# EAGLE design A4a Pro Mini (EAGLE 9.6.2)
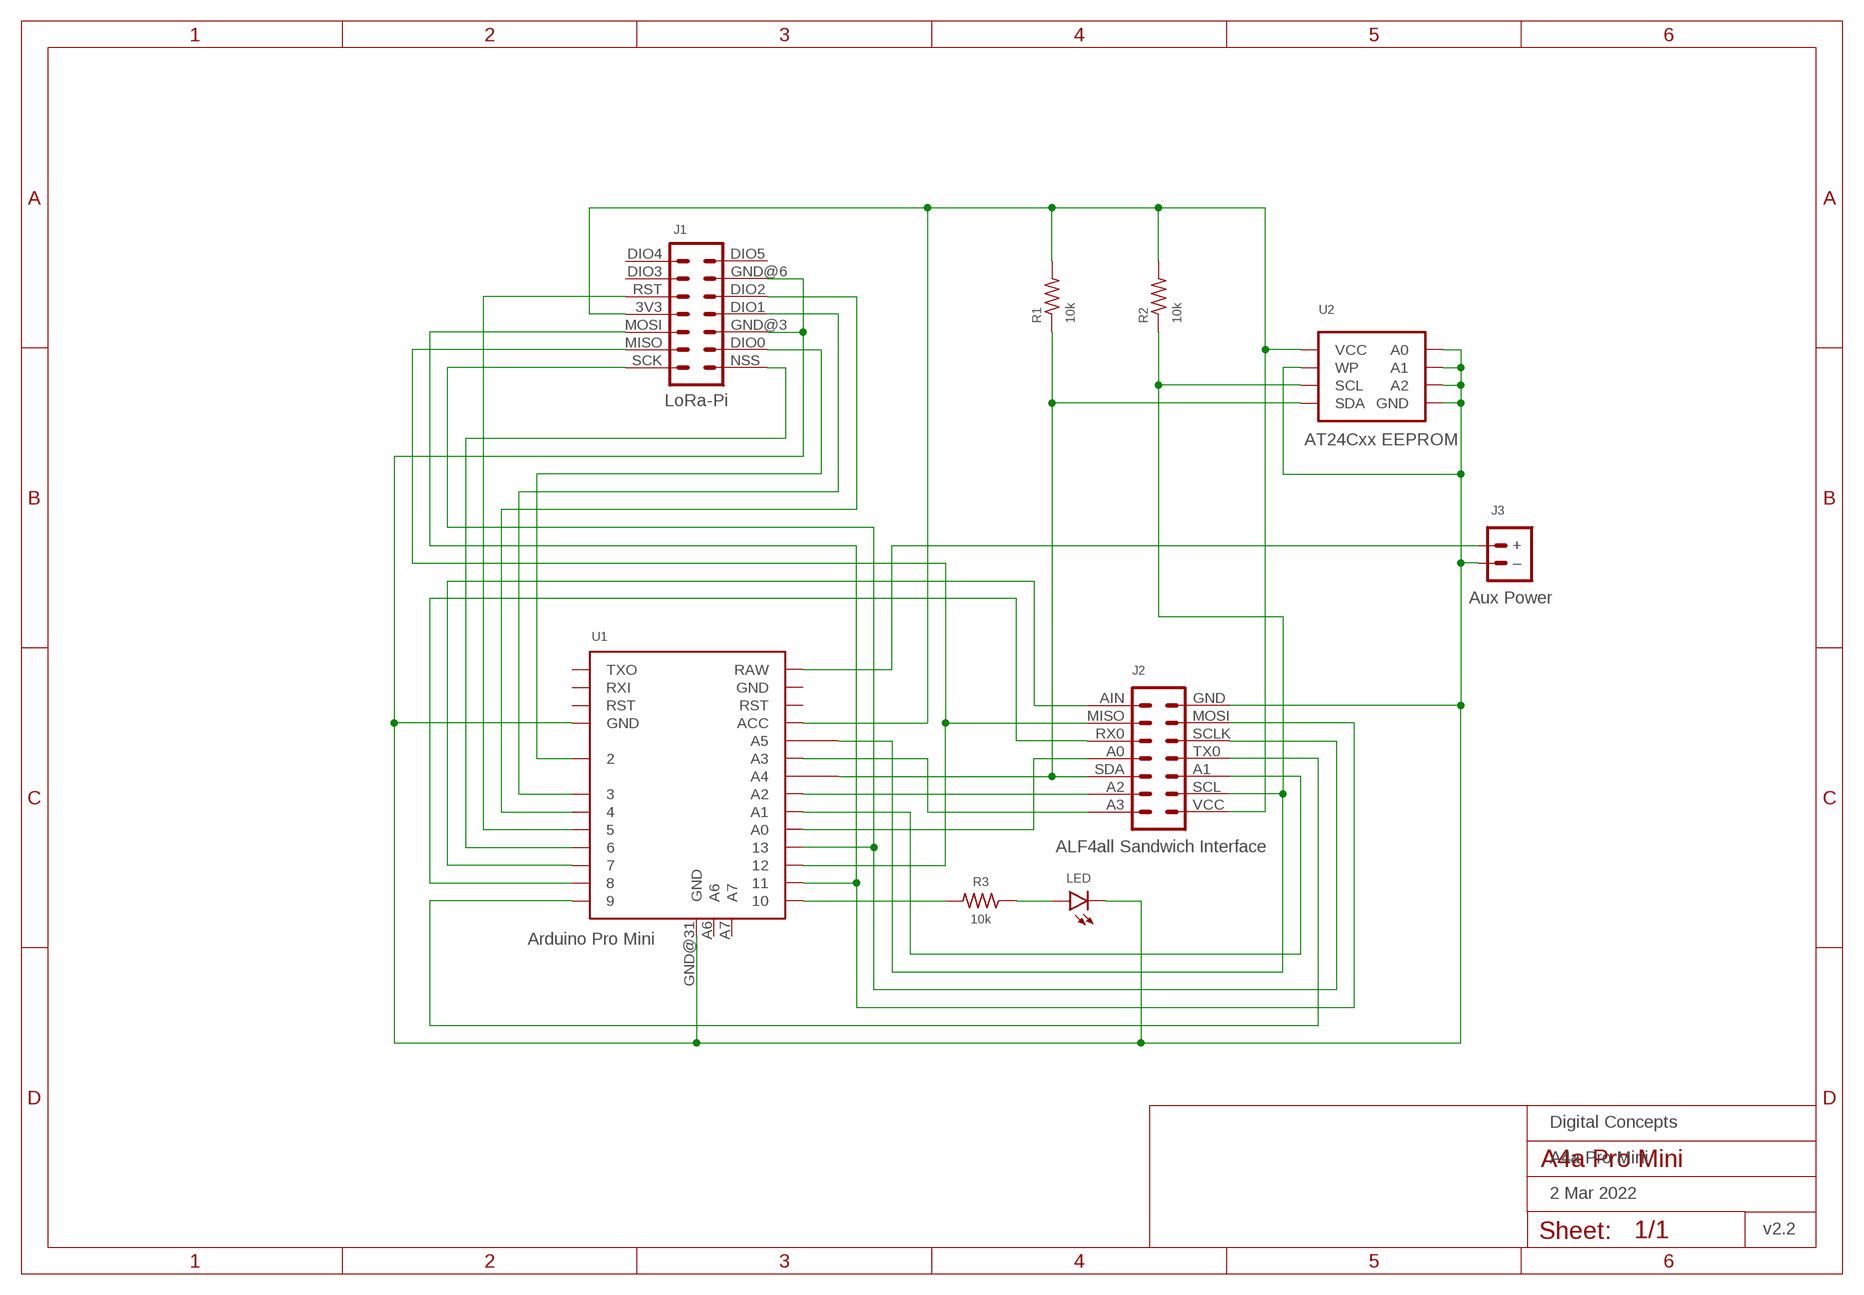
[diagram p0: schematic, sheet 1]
FRAME1 (A4L-LOC): DATE: 2 Mar 2022; OWNER: Digital Concepts; TITLE: A4a Pro Mini; VERSION: v2.2

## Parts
J1  LoRa-Pi  RFM95W-PI-HEADER  [RFM95W-PI]
J2  ALF4all Sandwich Interface  HEADER-2X7-ALF4ALL-PROCESSOR-B  [CONN_2X7-ALF4ALL-PROCESSOR-B]
J3  Aux Power  JST-PH2.0-2-MALE-HORIZONTALJST-PTH-2  [JST-PH2.0-2-HORIZONTAL]
LED  LEDCHIP-LED0805  [CHIP-LED0805]
R1  10k  RESISTORR0805  [R0805]
R2  10k  RESISTORR0805  [R0805]
R3  10k  RESISTORR0805  [R0805]
U1  Arduino Pro Mini  ARDUINO-PRO-MINI-35  [ARDUINO-PRO-MINI-35]
U2  AT24Cxx EEPROM  AT24CXX-EEPROM  [SOP-8]

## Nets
GND: J1.GND@3 J1.GND@6 J2.GND J3.-(–) LED.C U1.GND@22(GND) U1.GND@31(GND) U2.P$1(A0) U2.P$2(A1) U2.P$3(A2) U2.P$4(GND) U2.P$7(WP)
N$1: J2.A0 U1.A0
N$2: J2.A1 U1.A1
N$3: J2.A2 U1.A2
N$4: J2.A3 U1.A3
N$5: J3.+ U1.RAW
N$6: J1.SCK J2.SCLK U1.13
N$7: J2.RX0 U1.8
N$9: J2.AIN U1.7
N$10: J2.SDA R1.1 U1.A4 U2.P$5(SDA)
N$11: J2.SCL R2.1 U1.A5 U2.P$6(SCL)
N$12: J1.MISO J2.MISO U1.12
N$13: J1.MOSI J2.MOSI U1.11
N$14: J2.TX0 U1.9
N$15: J1.NSS U1.6
N$16: J1.RST U1.5
N$17: J1.DIO2 U1.4
N$18: J1.DIO1 U1.3
N$19: J1.DIO0 U1.2
N$20: R3.2 U1.10
N$21: LED.A R3.1
VCC: J1.3V3 J2.VCC R1.2 R2.2 U1.ACC U2.P$8(VCC)
Unconnected: J1.DIO3 J1.DIO4 J1.DIO5 U1.A6 U1.A7 U1.GND@11(GND) U1.RST@10(RST) U1.RST@21(RST) U1.RXI@20(RXI) U1.TXO@19(TXO)

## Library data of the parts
J1 = digitalconcepts:RFM95W-PI-HEADER: RFM95W LoRa Wireless Transceiver Raspberry Pi Daughter Board
J2 = digitalconcepts:HEADER-2X7-ALF4ALL-PROCESSOR-B: ALF4all 'Sandwich' Processor (Bottom) 2x7 Pin Header Header soldered to underside of PCB
J3 = digitalconcepts:JST-PH2.0-2-MALE-HORIZONTAL: Multi connection point. Often used as Generic Header-pin footprint for 0.1 inch spaced/style header connections; PROD_ID: CONN-09863; SKU: PRT-09914
LED = digitalconcepts:LED: LED
R1-R3 = digitalconcepts:RESISTOR: Resistor; SPICEPREFIX: R
U1 = digitalconcepts:ARDUINO-PRO-MINI-35: Arduino Pro Mini 35-pin Clone
U2 = digitalconcepts:AT24CXX-EEPROM: AT24Cxx EEPROM SOP-8

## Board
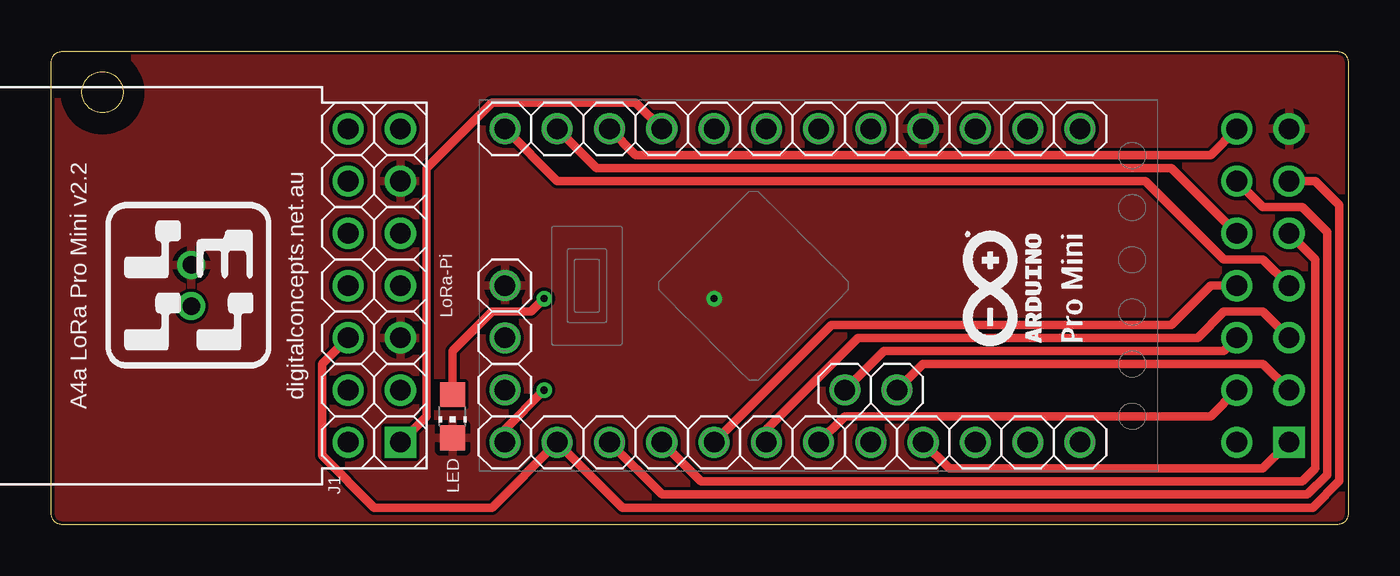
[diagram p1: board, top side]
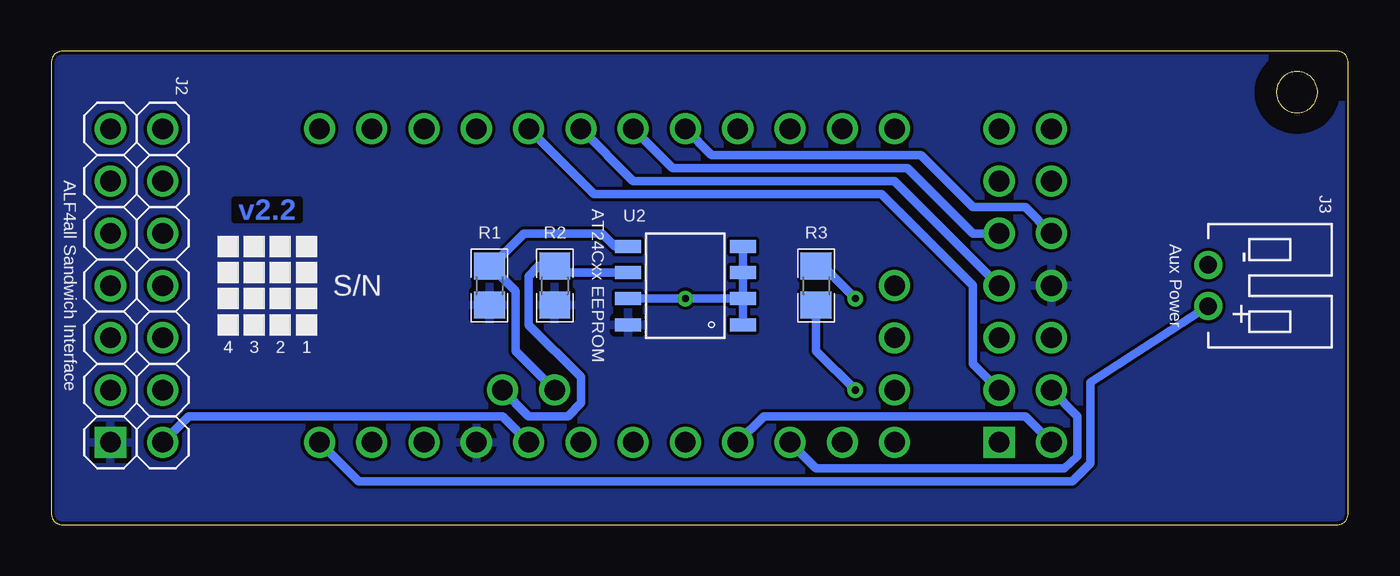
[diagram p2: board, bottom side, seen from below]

Size 63 x 23 mm. Coordinates in mm from the lower left corner, seen from the top.
Outline: 179 segments
Copper layers (1*16): Top 0.035mm / dielectric 1.5mm / Bottom 0.035mm
Design rules "default *": minimum track width 6mil, minimum drill 0.35mm, track to track 6mil, track to pad 6mil, pad to pad 6mil, via to via 6mil, smd to smd 6mil, copper to edge 6mil, drill to drill 6mil, minimum pad ring 10mil, minimum via ring 8mil, stop-mask expansion 4mil, vias tented up to drill 0mil, thermal gap 10mil

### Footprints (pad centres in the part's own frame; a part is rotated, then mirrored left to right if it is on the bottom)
RFM95W-PI = drill 1 pad 1.524: 3V3 7.62,2.54; DIO0 2.54,0; DIO1 7.62,0; DIO2 10.16,0; DIO3 12.7,2.54; DIO4 15.24,2.54; DIO5 15.24,0; GND@3 5.08,0; GND@6 12.7,0; MISO 2.54,2.54; MOSI 5.08,2.54; RST 10.16,2.54; SCK 0,2.54 | drill 1 pad 1.524 square: NSS 0,0
CONN_2X7-ALF4ALL-PROCESSOR-B = drill 1 pad 1.524: A0 7.62,2.54; A1 5.08,0; A2 2.54,2.54; A3 0,2.54; AIN 15.24,2.54; GND 15.24,0; MISO 12.7,2.54; MOSI 12.7,0; RX0 10.16,2.54; SCL 2.54,0; SCLK 10.16,0; SDA 5.08,2.54; TX0 7.62,0 | drill 1 pad 1.524 square: VCC 0,0
JST-PH2.0-2-HORIZONTAL = drill 0.85: + 1,0; - -1,0
CHIP-LED0805 = smd 1.2 x 1.2: A 0,-1.05; C 0,1.05
R0805 = smd 1.3 x 1.5: 1 -0.95,0; 2 0.95,0
ARDUINO-PRO-MINI-35 = drill 1: 2 -15.24,17.78; 3 -15.24,15.24; 4 -15.24,12.7; 5 -15.24,10.16; 6 -15.24,7.62; 7 -15.24,5.08; 8 -15.24,2.54; 9 -15.24,0; 10 0,0; 11 0,2.54; 12 0,5.08; 13 0,7.62; A0 0,10.16; A1 0,12.7; A2 0,15.24; A3 0,17.78; A4 -2.54,16.51; A5 -2.54,19.05; A6 -5.08,0; A7 -2.54,0; ACC 0,20.32; GND@11 0,25.4; GND@22 -15.24,20.32; GND@31 -7.62,0; RAW 0,27.94; RST@10 0,22.86; RST@21 -15.24,22.86; RXI@20 -15.24,25.4; TXO@19 -15.24,27.94
SOP-8 = smd 0.635 x 1.27: P$1 -1.905,-2.794; P$2 -0.635,-2.794; P$3 0.635,-2.794; P$4 1.905,-2.794; P$5 1.905,2.794; P$6 0.635,2.794; P$7 -0.635,2.794; P$8 -1.905,2.794

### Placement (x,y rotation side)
J1  16.96,4 90 top
J2  60.14,4 90 top
J3  6.8,11.62 270 bottom
LED  19.5,5.27 180 top
R1  41.72,11.62 270 bottom
R2  38.55,11.62 270 bottom
R3  25.85,11.62 270 bottom
U1  22.04,4 270 top
U2  32.2,11.62 90 bottom

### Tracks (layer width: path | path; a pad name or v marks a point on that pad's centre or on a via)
$X1
  cutout Top: 2.48,23.05 arc180 2.48,18.98 arc180
$X10
  cutout Bottom: 2.48,23.05 arc180 2.48,18.98 arc180
GND  (via drill 0.35)
  Bottom 0.406: U2.P$2 U2.P$3 U2.P$4 | U2.P$2 U2.P$1 | U2.P$2 v32.2,10.98 U2.P$7
  pour Top: -2.09,25.59 65.22,25.59 65.22,-2.35 -2.09,-2.35
N$1
  Top 0.406: J2.A0 56.33,11.62 54.42,9.71 37.91,9.71 U1.A0
N$2
  Top 0.406: J2.A1 58.87,10.35 56.96,10.35 55.69,9.08 39.18,9.08 34.74,4.63 U1.A1
N$3
  Top 0.406: J2.A2 56.33,5.27 38.55,5.27 U1.A2
N$4
  Bottom 0.406: J2.A3 56.33,5.27 41.09,5.27 U1.A3
N$5
  Bottom 0.406: J3.+ 12.51,6.9 12.51,2.98 13.4,2.09 48.07,2.09 U1.RAW
N$6
  Top 0.406: J2.SCLK 61.41,12.89 61.41,2.73 60.77,2.09 31.56,2.09 U1.13
  Bottom 0.406: J1.SCK 15.69,5.27 28.39,5.27 U1.13
N$7
  Top 0.406: J2.RX0 54.42,17.33 26.48,17.33 U1.8
N$9
  Top 0.406: J2.AIN 56.33,17.97 28.39,17.97 U1.7
N$10
  Top 0.406: J2.SDA 56.96,8.44 40.45,8.44 U1.A4
  Bottom 0.406: U2.P$5 35.62,13.52 36.26,14.16 40.03,14.16 41.62,12.57 R1.1 41.67,12.57 40.45,11.35 40.45,8.44 U1.A4
N$11
  Top 0.406: J2.SCL 58.87,7.81 42.36,7.81 U1.A5
  Bottom 0.406: U1.A5 39.82,5.27 37.91,5.27 37.28,5.9 37.28,7.17 39.82,9.71 39.82,12.07 39.33,12.57 R2.1 38.23,12.25 U2.P$6
N$12
  Top 0.406: J2.MISO 58.87,15.43 60.77,15.43 61.99,14.21 61.99,2.42 61.02,1.46 29.66,1.46 U1.12
  Bottom 0.406: J1.MISO 13.15,5.27 13.15,3.31 13.78,2.73 25.85,2.73 U1.12
N$13
  Top 0.406: J2.MOSI 61.41,16.7 62.57,15.53 62.57,2.12 61.28,0.82 27.75,0.82 U1.11 21.4,0.82 15.69,0.82 13.15,3.36 13.15,7.81 J1.MOSI
N$14
  Top 0.406: J2.TX0 58.87,12.89 56.96,12.89 53.15,16.7 24.58,16.7 U1.9
N$15
  Top 0.406: J1.NSS 18.23,5.27 18.23,17.33 21.4,20.51 28.39,20.51 U1.6
N$16
  Bottom 0.406: J1.RST 15.69,15.43 18.23,15.43 20.77,17.97 30.93,17.97 U1.5
N$17
  Bottom 0.406: U1.4 32.83,17.33 21.4,17.33 18.23,14.16 J1.DIO2
N$18
  Bottom 0.406: U1.3 34.74,16.7 22.04,16.7 J1.DIO1
N$19
  Bottom 0.406: U1.2 36.64,16.06 22.67,16.06 18.23,11.62 18.23,7.81 J1.DIO0
N$20  (via drill 0.35)
  Top 0.406: v23.94,6.54 22.04,4.63 U1.10
  Bottom 0.406: v23.94,6.54 25.85,8.44 R3.2
N$21  (via drill 0.35)
  Top 0.406: v23.94,10.98 23.3,10.35 21.4,10.35 19.5,8.44 LED.A
  Bottom 0.406: R3.1 25.53,12.57 v23.94,10.98
VCC
  Top 0.406: J2.VCC 58.87,2.73 43.63,2.73 U1.ACC
  pour Bottom: -0.82,24.32 63.95,24.32 63.95,-1.08 -0.82,-1.08

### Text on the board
Bottom: v2.2
tPlace: A4a LoRa Pro Mini v2.2 | digitalconcepts.net.au
bPlace: S/N | 1 | 2 | 3 | 4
